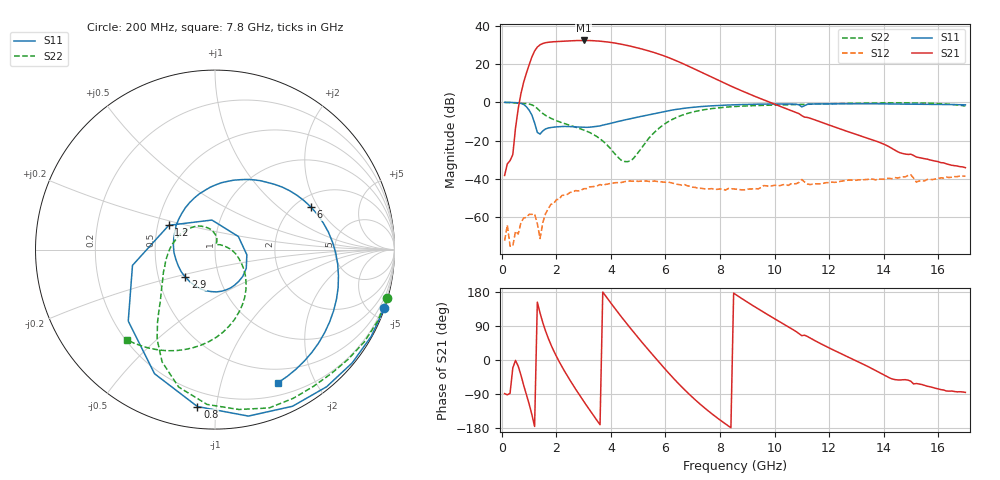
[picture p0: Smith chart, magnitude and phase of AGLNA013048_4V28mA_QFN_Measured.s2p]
! Filename4Jim: M058_Board_B02_0003_LRMTRL_NF2_NF.s2p
! Calibration: Board LRM+TRL, good to 17GHz
! Notes: Ray
! Row:0, Col:3
! Probes: nan
! Prober: MPI TS150
! Date: 2023-09-28 16:05:58
! DC: Vd.V=3.99994, Vd.I=0.0277489
! Keysight Technologies,N5245B,MY58421923,A.15.75.19
! AGMDC-PNAX50 Thu Sep 28 16:06:34 2023
# GHZ S DB R 50
!freq (Hz)  S11DB  S11A  S21DB  S21A  S12DB  S12A  S22DB  S22A
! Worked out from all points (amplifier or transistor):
!   170 points, 100 MHz to 17 GHz, reference 50 ohm
!   highest |S21| = 32.3 dB at 3 GHz (marker M1)
!   |S21| within 3 dB of that: 1.338 GHz to 4.723 GHz (3.385 GHz wide, 112 % of centre)
!   unconditionally stable (mu >= 1): 115 MHz to end of sweep
!   at 2.9 GHz: K = 2.24, MAG = 32.8 dB, |S12| = -45.8 dB
!   at 8.6 GHz: K = 4.12, MAG = 17.1 dB, |S12| = -45.3 dB
!   at 17 GHz: K = 192.04, MAG = -23.6 dB, |S12| = -38.5 dB
!   lowest NFmin = 0.58 dB at 3.6 GHz
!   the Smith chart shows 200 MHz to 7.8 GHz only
!   S11 on the Smith chart (normalised r, x): 200 MHz: 0.04, -5.95; 800 MHz: 0.11, -0.89; 1.2 GHz: 0.57, +0.17; 2.9 GHz: 0.69, -0.22; 6 GHz: 2.42, +1.74; 7.8 GHz: 0.34, -1.53
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0.1  -0.01 -9.5  -38.08 -88.8  -72.10 -34.7  -0.01 -7.8
0.2  -0.02 -19.1  -32.03 -91.8  -63.95 -169.3  -0.03 -15.7
0.8  -1.11 -96.4  10.59 -67.0  -60.29 -151.5  -0.57 -62.2
1.1  -6.59 -169.2  23.65 -143.9  -58.37 116.4  -1.27 -92.9
1.2  -10.72 152.3  26.77 -175.5  -58.18 79.7  -2.03 -104.8
1.4  -16.52 29.4  30.01 124.0  -70.96 -24.1  -4.53 -122.9
1.6  -13.85 -30.8  31.09 77.0  -58.07 -155.2  -6.76 -132.8
2  -12.75 -67.5  31.69 9.7  -50.68 144.7  -9.57 -151.0
2.5  -12.57 -102.8  32.09 -53.6  -46.93 101.1  -11.97 179.1
2.9  -12.93 -137.3  32.26 -98.1  -45.84 79.6  -13.90 150.5
3  -12.96 -146.7  32.28 -108.8  -45.02 77.0  -14.46 143.4
3.6  -12.25 156.3  31.90 -170.8  -42.84 41.2  -19.00 100.0
4  -10.87 125.1  31.25 150.0  -42.20 25.5  -24.36 80.0
4.4  -9.51 99.8  30.26 112.3  -41.73 6.5  -30.39 76.5
5.1  -7.34 65.5  27.96 50.1  -41.03 -32.1  -24.27 16.1
5.8  -5.23 33.6  24.97 -8.9  -41.35 -70.3  -13.05 -40.5
6  -4.65 23.8  23.95 -25.1  -41.62 -80.1  -10.97 -52.5
7.8  -1.72 -64.7  12.42 -147.5  -45.35 -160.7  -3.06 -134.4
8.6  -1.22 -95.8  7.23 171.6  -45.26 168.0  -2.11 -162.4
11.4  -0.82 175.5  -8.72 54.3  -42.63 62.0  -0.94 110.0
14.2  -0.80 76.5  -23.11 -46.5  -39.57 -10.2  -0.27 68.0
17  -1.29 2.8  -34.05 -85.5  -38.45 -73.8  -1.89 4.0
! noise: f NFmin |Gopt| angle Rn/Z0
0.8  4.627  0  90  0.4755
1.7  1.108  0  90  0.07264
2.7  0.709  0.1592  21.92  0.1525
3.7  0.6233  0.2651  34.23  0.1238
4.6  0.6875  0  90  0.04288
5.6  0.8786  0  90  0.05606
6.6  0.9297  0.3357  35.06  0.2022
7.5  1.515  0  90  0.1043
8.5  1.392  0.5167  119.6  0.1441
9.5  4.294  0  90  0.4219
